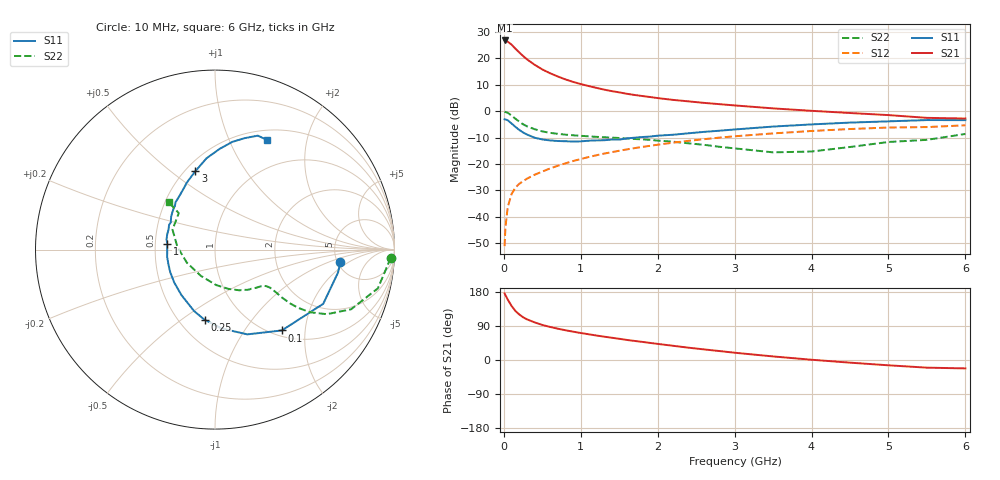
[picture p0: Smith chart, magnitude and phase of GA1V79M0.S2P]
! Infineon Technologies  Discrete & RF Semiconductors
! BF775
! Si NPN RF Bipolar Junction Transistor in SOT23
! VCE = 1.75 V  IC = 9 mA
! Common Emitter S-Parameters:  May  1996
# GHz  S  MA  R  50
!  f  S11  S21  S12  S22
! GHz  MAG  ANG  MAG  ANG  MAG  ANG  MAG  ANG
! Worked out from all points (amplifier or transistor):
!   36 points, 10 MHz to 6 GHz, reference 50 ohm
!   highest |S21| = 26.7 dB at 10 MHz (marker M1)
!   |S21| within 3 dB of that: start of sweep to 146.6 MHz
!   unconditionally stable (mu >= 1): 551.4 MHz to 3.999 GHz; 5.409 GHz to 5.655 GHz
!   at 250 MHz: K = 0.68, MSG = 23.7 dB, |S12| = -26.5 dB
!   at 1.4 GHz: K = 1.14, MAG = 9.3 dB, |S12| = -15.5 dB
!   at 6 GHz: K = 0.99, MSG = 1.3 dB, |S12| = -5.4 dB
!   S11 on the Smith chart (normalised r, x): 10 MHz: 5.30, -1.46; 100 MHz: 1.10, -1.51; 250 MHz: 0.66, -0.61; 1 GHz: 0.58, +0.04; 3 GHz: 0.56, +0.61; 6 GHz: 0.62, +1.39
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0.01  0.702 -5.7  21.7 175.8  0.0028 89.7  0.9797 -2.7
0.02  0.6972 -10.6  21.36 171.4  0.0062 86.1  0.9636 -5.6
0.05  0.6743 -26.6  20.61 159.6  0.0152 79.0  0.9326 -13.4
0.1  0.5845 -50.4  18.11 142.8  0.027 68.5  0.8277 -23.7
0.15  0.5055 -69.1  15.18 129.5  0.0358 62.8  0.7197 -30.0
0.2  0.4413 -85.1  12.91 120.2  0.0423 60.2  0.6344 -33.4
0.25  0.3951 -98.5  11.05 112.8  0.0473 59.0  0.5655 -35.0
0.3  0.3617 -108.8  9.569 107.4  0.0528 59.3  0.5177 -35.6
0.4  0.3146 -126.6  7.528 99.3  0.0628 59.5  0.4554 -35.6
0.5  0.2915 -141.4  6.147 92.5  0.0721 60.7  0.4141 -35.0
0.6  0.2797 -152.9  5.214 87.3  0.0824 61.6  0.3891 -34.8
0.7  0.2725 -161.9  4.533 82.7  0.0927 62.1  0.3728 -34.7
0.8  0.2699 -171.2  3.983 78.5  0.103 61.8  0.3596 -35.1
1  0.2684 173.1  3.251 71.2  0.1243 61.7  0.3417 -36.3
1.1  0.2758 168.1  2.989 68.0  0.1354 61.2  0.3344 -37.7
1.6  0.3056 143.1  2.128 52.9  0.1892 57.6  0.3033 -45.3
2.2  0.3581 123.7  1.632 37.5  0.2535 51.4  0.2646 -59.0
3  0.4503 104.1  1.283 19.2  0.3348 41.2  0.1978 -88.0
3.5  0.511 95.3  1.128 9.4  0.3796 34.5  0.1663 -118.1
4.5  0.6075 80.9  0.922 -7.0  0.4593 20.9  0.21 176.0
5.5  0.6782 69.4  0.747 -20.2  0.4997 6.7  0.2867 134.8
6  0.6761 64.5  0.725 -22.2  0.5401 2.7  0.3705 134.2
